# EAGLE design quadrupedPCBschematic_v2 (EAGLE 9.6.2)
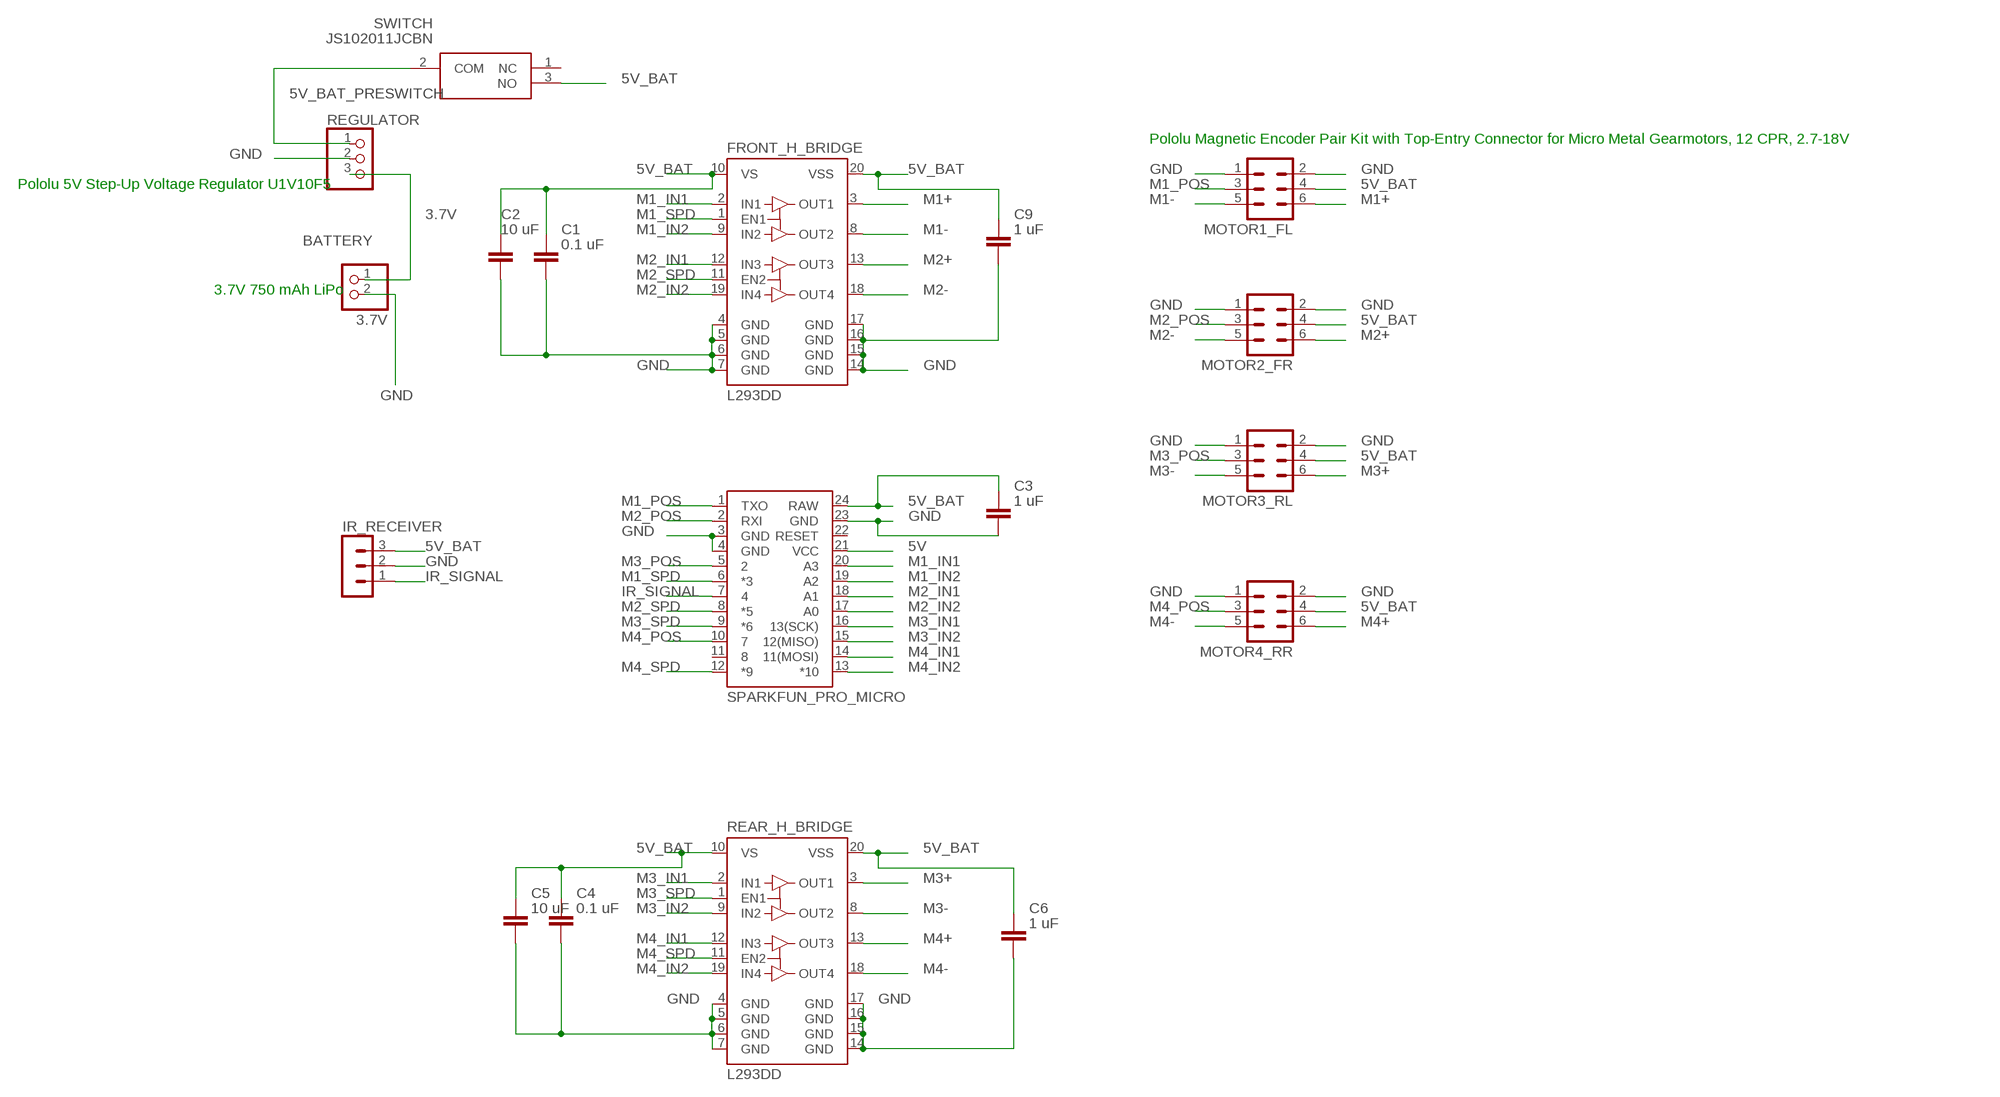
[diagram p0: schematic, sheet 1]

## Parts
B1  SPARKFUN_PRO_MICRO  [SPARKFUN_PRO_MICRO]
BATTERY  3.7V  PINHD-1X2  [1X02]
C1  0.1 uF  C_CHIP-0603(1608-METRIC)  [CAPC1608X85]
C2  10 uF  C_CHIP-0603(1608-METRIC)  [CAPC1608X85]
C3  1 uF  C_CHIP-0603(1608-METRIC)  [CAPC1608X85]
C4  0.1 uF  C_CHIP-0603(1608-METRIC)  [CAPC1608X85]
C5  10 uF  C_CHIP-0603(1608-METRIC)  [CAPC1608X85]
C6  1 uF  C_CHIP-0603(1608-METRIC)  [CAPC1608X85]
C9  1 uF  C_CHIP-0603(1608-METRIC)  [CAPC1608X85]
FRONT_H_BRIDGE  L293DD  [SO20]
IR_RECEIVER  MA03-1  [MA03-1]
MOTOR1_FL  MA03-2  [MA03-2]
MOTOR2_FR  MA03-2  [MA03-2]
MOTOR3_RL  MA03-2  [MA03-2]
MOTOR4_RR  MA03-2  [MA03-2]
REAR_H_BRIDGE  L293DD  [SO20]
REGULATOR  PINHD-1X3  [1X03]
SWITCH  JS102011JCBN  [JS102011JCBN]

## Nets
3.7V [high_V]: BATTERY.1 REGULATOR.3
5V: B1.21(VCC)
5V_BAT [high_V]: B1.24(RAW) C1.1 C2.1 C3.1 C4.1 C5.1 C6.1 C9.1 FRONT_H_BRIDGE.10(VS) FRONT_H_BRIDGE.20(VSS) IR_RECEIVER.3 MOTOR1_FL.4 MOTOR2_FR.4 MOTOR3_RL.4 MOTOR4_RR.4 REAR_H_BRIDGE.10(VS) REAR_H_BRIDGE.20(VSS) SWITCH.3(NO)
5V_BAT_PRESWITCH [high_V]: REGULATOR.1 SWITCH.2(COM)
GND [high_V]: B1.3(GND) B1.4(GND) B1.23(GND) BATTERY.2 C1.2 C2.2 C3.2 C4.2 C5.2 C6.2 C9.2 FRONT_H_BRIDGE.4(GND) FRONT_H_BRIDGE.5(GND) FRONT_H_BRIDGE.6(GND) FRONT_H_BRIDGE.7(GND) FRONT_H_BRIDGE.14(GND) FRONT_H_BRIDGE.15(GND) FRONT_H_BRIDGE.16(GND) FRONT_H_BRIDGE.17(GND) IR_RECEIVER.2 MOTOR1_FL.1 MOTOR1_FL.2 MOTOR2_FR.1 MOTOR2_FR.2 MOTOR3_RL.1 MOTOR3_RL.2 MOTOR4_RR.1 MOTOR4_RR.2 REAR_H_BRIDGE.4(GND) REAR_H_BRIDGE.5(GND) REAR_H_BRIDGE.6(GND) REAR_H_BRIDGE.7(GND) REAR_H_BRIDGE.14(GND) REAR_H_BRIDGE.15(GND) REAR_H_BRIDGE.16(GND) REAR_H_BRIDGE.17(GND) REGULATOR.2
IR_SIGNAL: B1.7 IR_RECEIVER.1
M1+: FRONT_H_BRIDGE.3(OUT1) MOTOR1_FL.6
M1-: FRONT_H_BRIDGE.8(OUT2) MOTOR1_FL.5
M1_IN1: B1.20(A3) FRONT_H_BRIDGE.2(IN1)
M1_IN2: B1.19(A2) FRONT_H_BRIDGE.9(IN2)
M1_POS: B1.1(TXO) MOTOR1_FL.3
M1_SPD: B1.6(*3) FRONT_H_BRIDGE.1(EN1)
M2+: FRONT_H_BRIDGE.13(OUT3) MOTOR2_FR.6
M2-: FRONT_H_BRIDGE.18(OUT4) MOTOR2_FR.5
M2_IN1: B1.18(A1) FRONT_H_BRIDGE.12(IN3)
M2_IN2: B1.17(A0) FRONT_H_BRIDGE.19(IN4)
M2_POS: B1.2(RXI) MOTOR2_FR.3
M2_SPD: B1.8(*5) FRONT_H_BRIDGE.11(EN2)
M3+: MOTOR3_RL.6 REAR_H_BRIDGE.3(OUT1)
M3-: MOTOR3_RL.5 REAR_H_BRIDGE.8(OUT2)
M3_IN1: B1.16(13(SCK)) REAR_H_BRIDGE.2(IN1)
M3_IN2: B1.15(12(MISO)) REAR_H_BRIDGE.9(IN2)
M3_POS: B1.5 MOTOR3_RL.3
M3_SPD: B1.9(*6) REAR_H_BRIDGE.1(EN1)
M4+: MOTOR4_RR.6 REAR_H_BRIDGE.13(OUT3)
M4-: MOTOR4_RR.5 REAR_H_BRIDGE.18(OUT4)
M4_IN1: B1.14(11(MOSI)) REAR_H_BRIDGE.12(IN3)
M4_IN2: B1.13(*10) REAR_H_BRIDGE.19(IN4)
M4_POS: B1.10 MOTOR4_RR.3
M4_SPD: B1.12(*9) REAR_H_BRIDGE.11(EN2)
Unconnected: B1.11 B1.22(RESET) SWITCH.1(NC)

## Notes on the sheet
- Pololu Magnetic Encoder Pair Kit with Top-Entry Connector for Micro Metal Gearmotors, 12 CPR, 2.7-18V
- Pololu 5V Step-Up Voltage Regulator U1V10F5
- 3.7V 750 mAh LiPo

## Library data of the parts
B1 = SparkFun-Boards:SPARKFUN_PRO_MICRO: SparkFun Pro Micro Atmega32U4 compatible footprint. SparkFun Products: 3.3V/8MHz 5V/16MHz
BATTERY = pinhead:PINHD-1X2: PIN HEADER
C1-C6 C9 = Capacitor:C: Capacitor - Generic; CATEGORY: Capacitor
FRONT_H_BRIDGE REAR_H_BRIDGE = st-microelectronics:L293DD: PUSH-PULL FOUR CHANNEL DRIVER WITH DIODES Source: http://www.st.com/stonline/books/pdf/docs/1330.pdf; OC_FARNELL: unknown
IR_RECEIVER = con-lstb:MA03-1: PIN HEADER; OC_FARNELL: unknown; OC_NEWARK: unknown
MOTOR1_FL MOTOR2_FR MOTOR3_RL MOTOR4_RR = con-lstb:MA03-2: PIN HEADER; OC_FARNELL: unknown; OC_NEWARK: unknown
REGULATOR = pinhead:PINHD-1X3: PIN HEADER
SWITCH = SamacSys_Parts:JS102011JCBN: Slide Switches SWITCH SLIDE VERTICAL MOUNT J BEND Source: Datasheet; ARROW_PART_NUMBER: JS102011JCBN; ARROW_PRICE-STOCK: https://www.arrow.com/en/products/js102011jcbn/ck?region=europe; DESCRIPTION: Slide Switches SWITCH SLIDE VERTICAL MOUNT J BEND; HEIGHT: 5.65mm; MANUFACTURER_NAME: C & K COMPONENTS; MANUFACTURER_PART_NUMBER: JS102011JCBN; MOUSER_PART_NUMBER: 611-JS102011JCBN; MOUSER_PRICE-STOCK: https://www.mouser.co.uk/ProductDetail/CK/JS102011JCBN?qs=By6Nw2ByBD26VYrGngqYVg%3D%3D

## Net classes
0 default: width 0.254 mm, drill 0.254 mm, clearance 0.254 mm
1 high_V: width 0.381 mm, drill 0.381 mm, clearance 0.381 mm

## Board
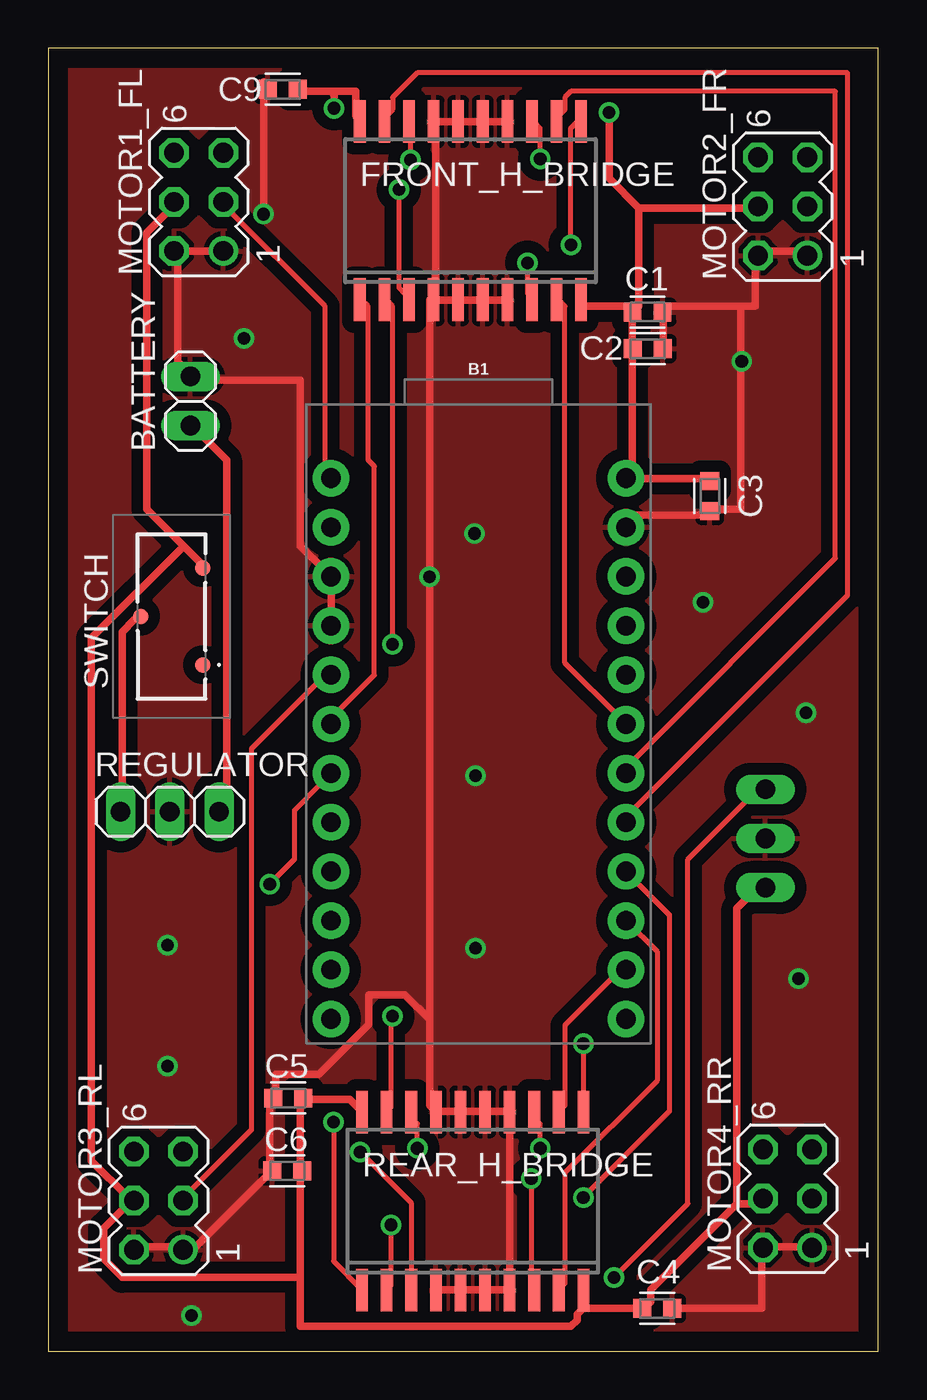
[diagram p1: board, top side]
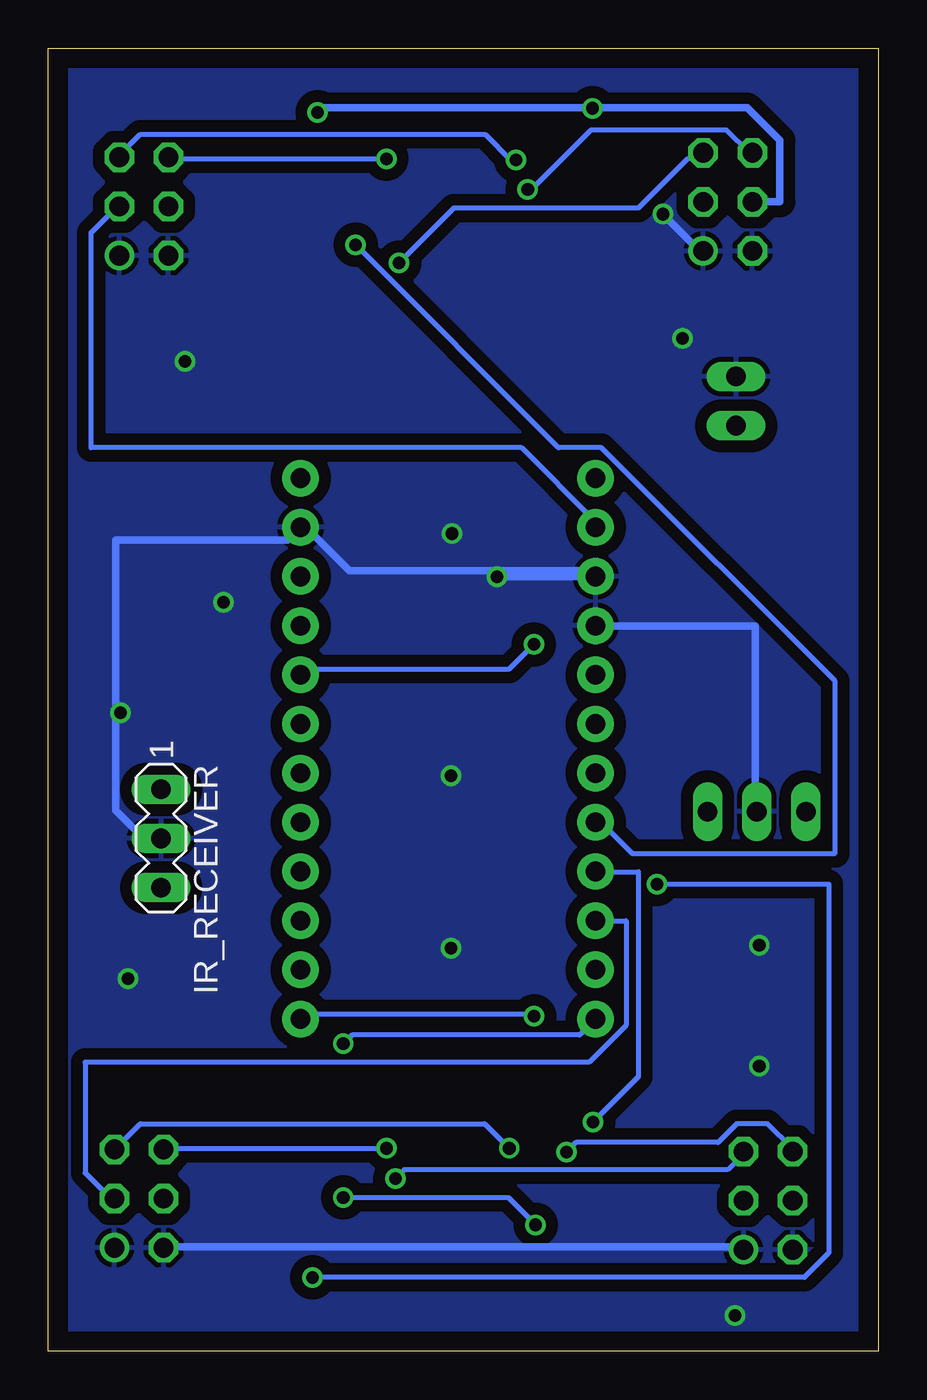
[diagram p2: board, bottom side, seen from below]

Size 42.85 x 67.3 mm. Coordinates in mm from the lower left corner, seen from the top.
Outline: 0,0 42.85,0 42.85,67.3 0,67.3 0,0
Copper layers (1*16): Top 0.035mm / dielectric 1.5mm / Bottom 0.035mm
Design rules "default *": minimum track width 6mil, minimum drill 0.35mm, track to track 6mil, track to pad 6mil, pad to pad 6mil, via to via 6mil, smd to smd 6mil, copper to edge 40mil, drill to drill 6mil, minimum pad ring 10mil, minimum via ring 8mil, stop-mask expansion 4mil, vias tented up to drill 0mil, thermal gap 10mil

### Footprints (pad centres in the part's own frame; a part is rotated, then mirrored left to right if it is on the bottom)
SPARKFUN_PRO_MICRO = drill 1.016 pad 1.88: 1 -7.62,12.7; 2 -7.62,10.16; 3 -7.62,7.62; 4 -7.62,5.08; 5 -7.62,2.54; 6 -7.62,0; 7 -7.62,-2.54; 8 -7.62,-5.08; 9 -7.62,-7.62; 10 -7.62,-10.16; 11 -7.62,-12.7; 12 -7.62,-15.24; 13 7.62,-15.24; 14 7.62,-12.7; 15 7.62,-10.16; 16 7.62,-7.62; 17 7.62,-5.08; 18 7.62,-2.54; 19 7.62,0; 20 7.62,2.54; 21 7.62,5.08; 22 7.62,7.62; 23 7.62,10.16; 24 7.62,12.7
1X02 = drill 1.016 long: 1 -1.27,0; 2 1.27,0
CAPC1608X85 = smd 0.921 x 0.97: 1 -0.775,0; 2 0.775,0
SO20 = smd 0.6 x 2.2: 1 -5.715,-4.6; 2 -4.445,-4.6; 3 -3.175,-4.6; 4 -1.905,-4.6; 5 -0.635,-4.6; 6 0.635,-4.6; 7 1.905,-4.6; 8 3.175,-4.6; 9 4.445,-4.6; 10 5.715,-4.6; 11 5.715,4.6; 12 4.445,4.6; 13 3.175,4.6; 14 1.905,4.6; 15 0.635,4.6; 16 -0.635,4.6; 17 -1.905,4.6; 18 -3.175,4.6; 19 -4.445,4.6; 20 -5.715,4.6
MA03-1 = drill 1.016 long: 1 -2.54,0; 2 0,0; 3 2.54,0
MA03-2 = drill 1.016: 1 -2.54,-1.27 | drill 1.016 octagon: 2 -2.54,1.27; 3 0,-1.27; 4 0,1.27; 5 2.54,-1.27; 6 2.54,1.27
1X03 = drill 1.016 long: 1 -2.54,0; 2 0,0; 3 2.54,0
JS102011JCBN = smd 0.8 x 0.8: 1 -2.5,-1.6; 2 0,1.6; 3 2.5,-1.6

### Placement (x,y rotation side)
B1  22.21,32.4 0 top
BATTERY  7.33,49.08 90 top
C1  30.94,53.68 0 top
C2  30.96,51.78 0 top
C3  34.16,44.18 270 top
C4  31.44,2.21 0 top
C5  12.39,13.07 180 top
C6  12.33,9.31 180 top
C9  12.11,65.18 180 top
FRONT_H_BRIDGE  21.8,58.92 0 top
IR_RECEIVER  37.03,26.48 270 bottom
MOTOR1_FL  7.76,59.37 90 top
MOTOR2_FR  37.92,59.14 90 top
MOTOR3_RL  5.68,7.78 90 top
MOTOR4_RR  38.17,7.88 90 top
REAR_H_BRIDGE  21.91,7.75 0 top
REGULATOR  6.27,27.87 0 top
SWITCH  6.36,37.96 90 top

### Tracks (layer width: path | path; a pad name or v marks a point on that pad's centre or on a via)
3.7V
  Top 0.381: REGULATOR.3 8.89,27.94 9.21,28.26 9.21,46.04 7.62,47.62 BATTERY.1
5V_BAT  (via drill 0.65)
  Top 0.381: 27.62,2.22 30.48,2.22 C4.1 30.8,2.22 31.11,2.54 31.11,3.17 35.56,7.62 | 27.62,2.22 27.62,2.86 REAR_H_BRIDGE.10 27.62,2.22 | 35.56,7.62 36.83,7.62 MOTOR4_RR.4 | REAR_H_BRIDGE.20 16.19,12.38 15.56,13.02 13.34,13.02 C5.1 13.02,13.02 13.02,9.53 C6.1 13.02,9.21 13.02,3.81 | 13.02,3.81 3.81,3.81 2.86,4.76 2.86,6.35 4.13,7.62 MOTOR3_RL.4 4.13,7.94 2.22,9.84 2.22,36.83 6.99,41.59 | 27.62,2.22 27.3,1.91 27.3,1.59 26.99,1.27 13.02,1.27 13.02,3.81 | C3.1 33.97,45.09 29.84,45.09 B1.24 29.84,45.4 30.16,45.72 30.16,51.75 C2.1 30.16,52.07 30.16,53.66 C1.1 | C1.1 30.16,53.98 27.62,53.98 27.62,54.29 FRONT_H_BRIDGE.10 | 30.48,59.05 36.51,59.05 MOTOR2_FR.4 | 30.48,59.05 30.48,53.98 C1.1 | 14.75,65.09 15.88,65.09 15.88,63.82 FRONT_H_BRIDGE.20 | 14.75,65.09 13.15,65.09 C9.1 | 6.99,41.59 5.08,43.5 5.08,57.78 6.35,59.05 MOTOR1_FL.4 | 6.99,41.59 7.94,40.64 SWITCH.3 | v14.75,64.21 14.75,64.88 14.75,65.09 | 30.48,59.05 28.95,60.58 v28.95,64 | 35.56,7.62 35.56,22.86 36.83,24.13 IR_RECEIVER.3
  Bottom 0.381: MOTOR1_FL.4 6.35,59.37 5.08,59.37 5.08,62.55 6.77,64.23 14.72,64.23 v14.75,64.21 14.79,64.25 28.7,64.25 v28.95,64
5V_BAT_PRESWITCH
  Top 0.381: SWITCH.2 4.45,37.78 3.81,37.15 3.81,27.94 REGULATOR.1
GND  (via drill 0.65)
  Top 0.381: B1.23 29.84,42.86 29.84,43.18 33.97,43.18 C3.2 34.29,43.5 35.74,43.5 35.74,53.98 | C2.2 31.75,52.07 31.75,53.66 C1.2 31.75,53.98 35.74,53.98 | 35.74,53.98 36.51,53.98 36.51,56.52 MOTOR2_FR.2 36.83,56.83 39.05,56.83 MOTOR2_FR.1 | C9.2 11.11,65.57 v11.11,58.74 | MOTOR1_FL.1 8.89,56.83 6.67,56.83 MOTOR1_FL.2 6.67,56.52 6.67,51.12 7.3,50.48 BATTERY.2 7.62,50.16 13.02,50.16 13.02,41.59 14.29,40.32 B1.3 14.61,40.01 14.61,37.78 B1.4 | FRONT_H_BRIDGE.4 20,54.29 20.95,54.29 FRONT_H_BRIDGE.5 21.27,54.29 22.23,54.29 FRONT_H_BRIDGE.6 22.54,54.29 23.5,54.29 FRONT_H_BRIDGE.7 | 20,63.5 20.95,63.5 FRONT_H_BRIDGE.16 21.27,63.5 22.23,63.5 FRONT_H_BRIDGE.15 22.54,63.5 23.5,63.5 FRONT_H_BRIDGE.14 | 20,63.5 20,54.61 FRONT_H_BRIDGE.4 | 20,63.5 FRONT_H_BRIDGE.17 | 21.27,3.17 20,3.17 REAR_H_BRIDGE.4 | 21.27,3.17 22.54,3.17 | 21.27,3.17 REAR_H_BRIDGE.5 | 22.54,3.17 23.81,3.17 | 22.54,3.17 REAR_H_BRIDGE.6 | 21.27,12.38 20,12.38 | 21.27,12.38 22.54,12.38 | 21.27,12.38 REAR_H_BRIDGE.16 | 22.54,12.38 23.81,12.38 REAR_H_BRIDGE.14 23.81,12.06 23.81,3.17 | 22.54,12.38 REAR_H_BRIDGE.15 | 23.81,3.17 REAR_H_BRIDGE.7 | C4.2 32.38,2.22 36.83,2.22 36.83,5.08 MOTOR4_RR.2 37.15,5.4 39.37,5.4 MOTOR4_RR.1 | MOTOR3_RL.2 4.45,5.4 6.67,5.4 MOTOR3_RL.1 6.99,5.4 7.62,5.4 11.43,9.21 C6.2 11.43,9.53 11.43,13.02 C5.2 11.75,13.34 11.75,14.29 13.97,14.29 16.55,16.87 16.55,18.41 18.41,18.41 19.68,17.14 | 20,12.38 19.68,12.7 19.68,17.14 | 20,12.38 REAR_H_BRIDGE.17 | 19.68,17.14 v19.68,40.01 19.68,54.29 FRONT_H_BRIDGE.4
  Bottom 0.381: v11.11,58.74 9.21,56.83 MOTOR1_FL.1 | REGULATOR.2 6.35,27.94 6.35,37.47 14.29,37.47 B1.4 | MOTOR4_RR.2 36.83,5.4 6.99,5.4 MOTOR3_RL.1 | v19.68,40.01 14.61,40.01 B1.3 14.61,40.32 27.3,40.32 29.53,42.55 B1.23 30.48,41.91 39.37,41.91 39.37,27.94 38.1,26.67 IR_RECEIVER.2
  other vias: 35.81,51.13 10.11,52.33 22.01,42.24 33.81,38.69 22.06,29.72 39.12,32.98 6.14,20.97 6.14,14.73 7.39,1.85 22.06,20.81 38.74,19.24
  pour Top (isolate 0.61): 0.31,66.98 42.45,66.98 42.47,66.97 42.47,0.32 42.47,0.32 0.29,0.32 0.27,0.3 0.27,66.96 0.29,66.98
  pour Bottom (isolate 0.61): 0.28,67.15 42.64,67.15 42.64,0.14 42.64,0.14 0.14,0.14 0.14,0.14 0.14,67.06 0.22,67.15
IR_SIGNAL  (via drill 0.65)
  Top 0.254: v29.21,3.81 33.02,7.62 33.02,25.4 36.83,29.21 IR_RECEIVER.1 | v11.43,24.13 12.7,25.4 12.7,27.94 13.97,29.21 B1.7
  Bottom 0.254: v29.21,3.81 3.81,3.81 2.54,5.08 2.54,24.13 v11.43,24.13
M1+  (via drill 0.65)
  Top 0.254: v18.1,60.01 18.1,54.93 18.41,54.61 FRONT_H_BRIDGE.3
  Bottom 0.254: v18.1,60.01 17.91,60.01 14.84,63.08 7.83,63.08 6.67,61.91 MOTOR1_FL.6
M1-  (via drill 0.65)
  Top 0.254: v24.74,56.23 24.74,54.65 FRONT_H_BRIDGE.8
  Bottom 0.254: v24.74,56.23 21.91,59.05 12.38,59.05 9.84,61.59 9.21,61.59 MOTOR1_FL.5
M1_IN1  (via drill 0.65)
  Top 0.254: v17.78,36.51 17.78,53.98 17.46,54.29 FRONT_H_BRIDGE.2
  Bottom 0.254: v17.78,36.51 19.05,35.24 29.53,35.24 B1.20
M1_IN2
  Top 0.254: FRONT_H_BRIDGE.9 26.35,54.29 26.67,53.98 26.67,35.56 29.53,32.7 B1.19
M1_POS
  Top 0.254: MOTOR1_FL.3 9.21,59.05 14.29,53.98 14.29,45.4 B1.1
M1_SPD
  Top 0.254: FRONT_H_BRIDGE.1 16.19,54.29 16.51,53.98 16.51,46.04 16.83,45.72 16.83,34.92 14.61,32.7 B1.6
M2+  (via drill 0.65)
  Top 0.254: v25.4,61.59 25.4,63.18 25.08,63.5 FRONT_H_BRIDGE.13
  Bottom 0.254: v25.4,61.59 36.51,61.59 MOTOR2_FR.6
M2-  (via drill 0.65)
  Top 0.254: v18.7,61.53 18.7,63.51 FRONT_H_BRIDGE.18
  Bottom 0.254: v18.7,61.53 18.97,61.53 20.3,62.87 38.1,62.87 39.05,61.91 MOTOR2_FR.5
M2_IN1
  Top 0.254: FRONT_H_BRIDGE.12 26.35,63.82 26.67,64.14 26.67,64.77 26.99,65.09 40.64,65.09 40.64,40.96 29.84,30.16 B1.18
M2_IN2
  Top 0.254: FRONT_H_BRIDGE.19 17.46,63.82 17.78,64.14 17.78,64.77 19.05,66.04 41.27,66.04 41.27,39.05 29.84,27.62 B1.17
M2_POS
  Bottom 0.254: MOTOR2_FR.3 39.37,59.05 40.64,57.78 40.64,46.67 18.41,46.67 14.61,42.86 B1.2
M2_SPD  (via drill 0.65)
  Top 0.254: v26.99,57.15 26.99,63.18 27.3,63.5 FRONT_H_BRIDGE.11
  Bottom 0.254: v26.99,57.15 16.51,46.67 14.29,46.67 2.22,34.61 2.22,25.72 12.7,25.72 14.29,27.3 B1.8
M3+  (via drill 0.65)
  Top 0.254: v16.1,10.29 18.73,7.66 18.73,3.17 REAR_H_BRIDGE.3
  Bottom 0.254: v16.1,10.29 15.61,10.78 8.27,10.78 7.3,11.75 5.71,11.75 4.45,10.48 MOTOR3_RL.6
M3-  (via drill 0.65)
  Top 0.254: v24.93,8.91 24.93,3.32 25.08,3.17 REAR_H_BRIDGE.8
  Bottom 0.254: v24.93,8.91 24.48,9.37 7.78,9.37 6.99,10.16 MOTOR3_RL.5
M3_IN1  (via drill 0.65)
  Top 0.254: v17.69,6.52 17.69,3.4 17.46,3.17 REAR_H_BRIDGE.2 | v27.62,7.94 32.07,12.38 32.07,22.54 29.84,24.77 B1.16
  Bottom 0.254: v17.69,6.52 19.1,7.94 v27.62,7.94
M3_IN2
  Top 0.254: REAR_H_BRIDGE.9 26.35,3.17 26.67,3.49 26.67,9.21 31.43,13.97 31.43,20.64 29.84,22.23 B1.15
M3_POS
  Top 0.254: MOTOR3_RL.3 6.99,7.94 10.48,11.43 10.48,31.11 14.29,34.92 B1.5
M3_SPD  (via drill 0.65)
  Top 0.254: v14.72,11.84 14.72,4.64 16.19,3.17 REAR_H_BRIDGE.1
  Bottom 0.254: v14.72,11.84 12.38,14.18 12.38,24.77 14.29,24.77 B1.9
M4+  (via drill 0.65)
  Top 0.254: v25.4,10.48 25.4,11.75 25.08,12.06 REAR_H_BRIDGE.13
  Bottom 0.254: v25.4,10.48 36.83,10.48 MOTOR4_RR.6
M4-  (via drill 0.65)
  Top 0.254: v19.05,10.48 19.05,11.75 18.73,12.06 REAR_H_BRIDGE.18
  Bottom 0.254: v19.05,10.48 20.32,11.75 38.1,11.75 39.37,10.48 MOTOR4_RR.5
M4_IN1
  Top 0.254: REAR_H_BRIDGE.12 26.35,12.38 26.67,12.7 26.67,16.83 29.53,19.68 B1.14
M4_IN2  (via drill 0.65)
  Top 0.254: v17.76,17.3 17.69,17.3 17.69,12.61 17.46,12.38 REAR_H_BRIDGE.19
  Bottom 0.254: v17.76,17.3 17.88,17.42 29.57,17.42 B1.13
M4_POS
  Bottom 0.254: MOTOR4_RR.3 39.69,7.94 40.96,9.21 40.96,14.92 14.92,14.92 13.02,16.83 13.02,22.23 14.29,22.23 B1.10
M4_SPD  (via drill 0.65)
  Top 0.254: v27.62,15.88 27.62,12.38 REAR_H_BRIDGE.11
  Bottom 0.254: v27.62,15.88 27.16,16.33 15.42,16.33 14.61,17.14 B1.12
(copper drawn outside any net)
  shapes: Top area x1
